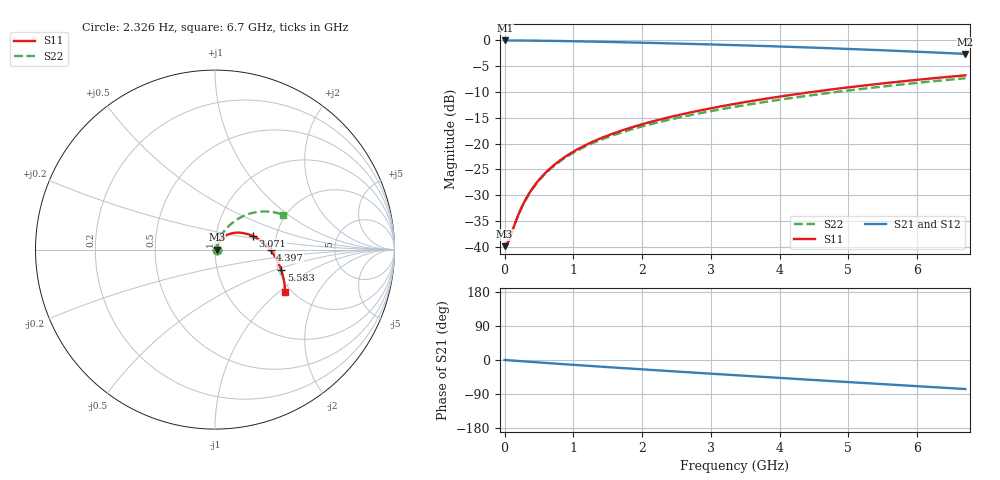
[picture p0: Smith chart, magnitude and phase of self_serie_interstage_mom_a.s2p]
! Created Mon Jan 20 16:22:58 2014
# ghz S ma R 50
! 2 Port Network Data from data block
! freq  magS11  angS11  magS21  angS21  magS12  angS12  magS22  angS22
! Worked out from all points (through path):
!   195 points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, 2.326 Hz to 6.7 GHz, reference 50 ohm
!   highest |S21| = -0.09 dB at 2.326 MHz (marker M1); lowest = -2.7 dB at 6.7 GHz (marker M2)
!   group delay of S21, straight-line fit = 31.7 ps
!   lowest |S11| = -39.8 dB at 2.326 Hz (marker M3), VSWR 1.02, Z = 51 + j1.98e-08 ohm
!   |S11| at or under -10 dB: start of sweep to 4.495 GHz
!   |S22| runs from -39.8 to -7.4 dB; largest |S21 - S12| = 0
!   S11 on the Smith chart (normalised r, x): 2.326 Hz: 1.02, +0.00; 3.071 GHz: 1.51, +0.24; 4.397 GHz: 1.90, -0.02; 5.583 GHz: 2.07, -0.55; 6.7 GHz: 1.86, -1.10
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2.326389e-09  0.01019 0.0  0.9898 -0.0  0.9898 -0.0  0.01019 0.0
0.002326389  0.01019 1.1  0.9898 -0.0  0.9898 -0.0  0.01019 1.1
0.02326389  0.0104 10.7  0.9898 -0.3  0.9898 -0.3  0.0104 10.9
0.04652778  0.01102 20.6  0.9897 -0.6  0.9897 -0.6  0.011 21.0
0.1861111  0.01949 52.3  0.9889 -2.5  0.9889 -2.5  0.01932 54.0
0.2791667  0.02676 58.7  0.9878 -3.7  0.9878 -3.7  0.02646 61.5
0.3722222  0.03426 61.3  0.9866 -4.9  0.9866 -4.9  0.03383 65.1
0.4594618  0.04132 61.9  0.9851 -6.0  0.9851 -6.0  0.04075 66.8
0.6048611  0.05298 61.4  0.9823 -7.9  0.9823 -7.9  0.05215 67.8
0.7502604  0.06443 59.7  0.9791 -9.7  0.9791 -9.7  0.06326 67.8
0.9247396  0.07784 57.1  0.9748 -11.9  0.9748 -11.9  0.07613 67.1
1.128299  0.09299 53.6  0.9692 -14.4  0.9692 -14.4  0.0905 66.0
1.360937  0.1097 49.4  0.9623 -17.2  0.9623 -17.2  0.1062 64.5
1.622656  0.128 44.7  0.9542 -20.3  0.9542 -20.3  0.123 62.7
2.268229  0.1712 33.2  0.9327 -27.8  0.9327 -27.8  0.1624 58.6
3.070833  0.2237 19.7  0.9033 -36.9  0.9033 -36.9  0.2098 53.6
3.384896  0.2441 14.7  0.8909 -40.4  0.8909 -40.4  0.2284 51.6
4.396875  0.3098 -0.7  0.8477 -51.7  0.8477 -51.7  0.2889 44.8
4.466667  0.3144 -1.7  0.8446 -52.5  0.8446 -52.5  0.2931 44.3
5.583333  0.3862 -17.1  0.7914 -64.6  0.7914 -64.6  0.3607 36.0
5.676389  0.3921 -18.3  0.7868 -65.6  0.7868 -65.6  0.3663 35.3
6.7  0.4558 -31.0  0.7339 -76.5  0.7339 -76.5  0.4274 27.0
